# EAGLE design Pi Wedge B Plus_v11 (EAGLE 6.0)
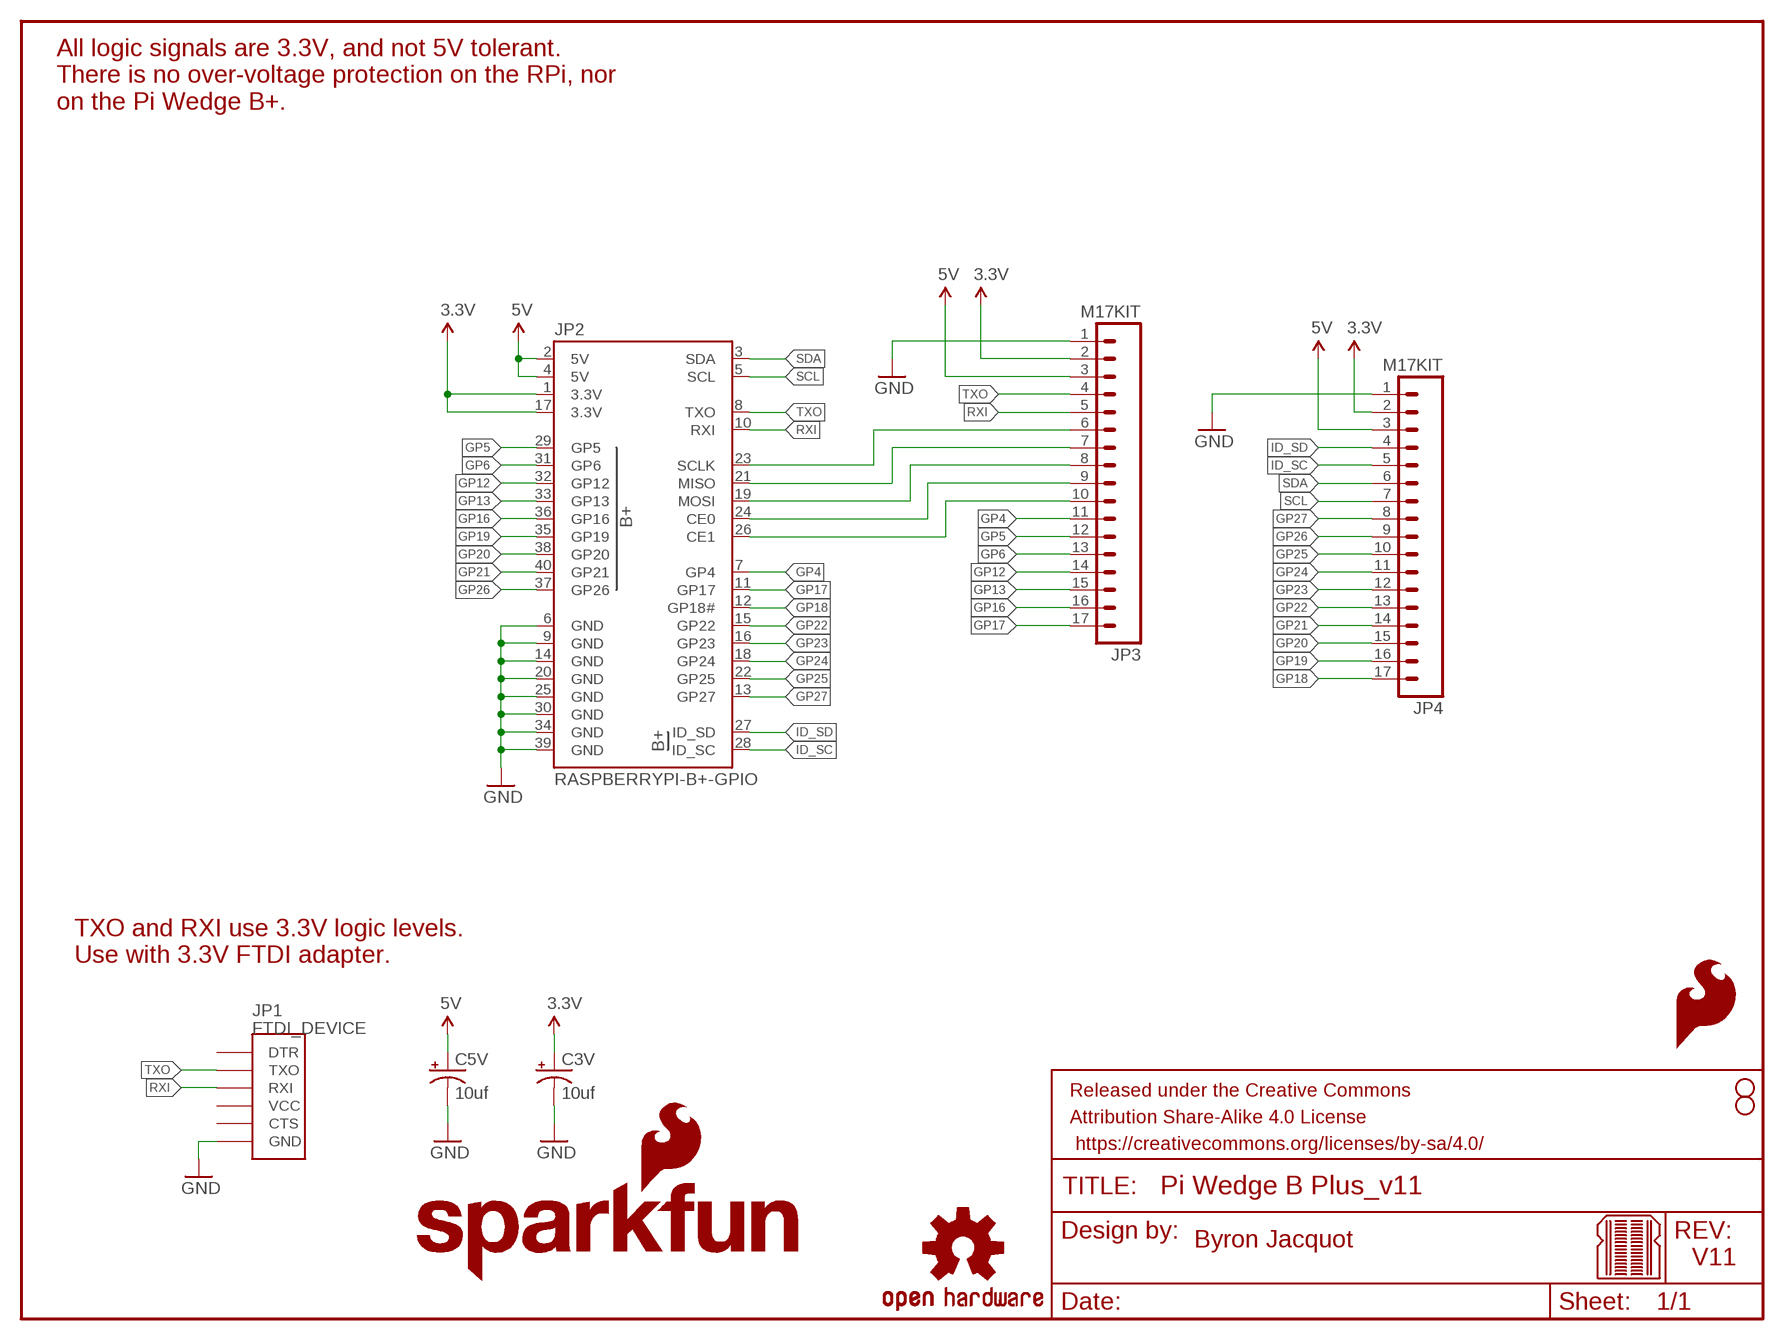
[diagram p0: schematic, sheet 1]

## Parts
C3V  10uf  10UF-25V-20%(PTH)KIT  [CPOL-RADIAL-10UF-25V-KIT]
C5V  10uf  10UF-25V-20%(PTH)KIT  [CPOL-RADIAL-10UF-25V-KIT]
FRAME2  FRAME-LETTER  [CREATIVE_COMMONS]
JP1  FTDI_DEVICE  [FTDI_DEVICE_SIDE]
JP2  RASPBERRYPI-B+-GPIO  [2X20-SHROUDED]
JP3  M17KIT  [1X17_NO_SILK_KIT]
JP4  M17KIT  [1X17_NO_SILK_KIT]
LOGO1  SFE_LOGO_NAME_FLAME.2_INCH  [SFE_LOGO_NAME_FLAME_.2]
LOGO2  SFE_LOGO_NAME_FLAME.2_INCH  [SFE_LOGO_NAME_FLAME_.2]
LOGO3  SFE_LOGO_FLAME.1_INCH  [SFE_LOGO_FLAME_.1]
LOGO4  SFE_LOGO_FLAME.1_INCH  [SFE_LOGO_FLAME_.1]
LOGO5  OSHW-LOGOS  [OSHW-LOGO-S]
STANDOFF1  STAND-OFF  [STAND-OFF]
STANDOFF2  STAND-OFF  [STAND-OFF]
U$2  BREADBOARD_PATTERN  [BREADBOARD_SPACING]

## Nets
3.3V: C3V.1(+) JP2.1(3.3V) JP2.17(3.3V) JP3.2 JP4.2
5V: C5V.1(+) JP2.2(5V) JP2.4(5V) JP3.3 JP4.3
CE0: JP2.24(CE0) JP3.9
CE1: JP2.26(CE1) JP3.10
GND: C3V.2(-) C5V.2(-) JP1.P$6(GND) JP2.6(GND) JP2.9(GND) JP2.14(GND) JP2.20(GND) JP2.25(GND) JP2.30(GND) JP2.34(GND) JP2.39(GND) JP3.1 JP4.1
GP4: JP2.7(GP4) JP3.11
GP5: JP2.29(GP5) JP3.12
GP6: JP2.31(GP6) JP3.13
GP12: JP2.32(GP12) JP3.14
GP13: JP2.33(GP13) JP3.15
GP16: JP2.36(GP16) JP3.16
GP17: JP2.11(GP17) JP3.17
GP18: JP2.12(GP18#) JP4.17
GP19: JP2.35(GP19) JP4.16
GP20: JP2.38(GP20) JP4.15
GP21: JP2.40(GP21) JP4.14
GP22: JP2.15(GP22) JP4.13
GP23: JP2.16(GP23) JP4.12
GP24: JP2.18(GP24) JP4.11
GP25: JP2.22(GP25) JP4.10
GP26: JP2.37(GP26) JP4.9
GP27: JP2.13(GP27) JP4.8
ID_SC: JP2.28(ID_SC) JP4.5
ID_SD: JP2.27(ID_SD) JP4.4
MISO: JP2.21(MISO) JP3.7
MOSI: JP2.19(MOSI) JP3.8
RXI: JP1.P$3(RXI) JP2.10(RXI) JP3.5
SCL: JP2.5(SCL) JP4.7
SCLK: JP2.23(SCLK) JP3.6
SDA: JP2.3(SDA) JP4.6
TXO: JP1.P$2(TXO) JP2.8(TXO) JP3.4
Unconnected: JP1.P$1(DTR) JP1.P$4(VCC) JP1.P$5(CTS)

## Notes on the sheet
- All logic signals are 3.3V, and not 5V tolerant.
  There is no over-voltage protection on the RPi, nor
  on the Pi Wedge B+.
- TXO and RXI use 3.3V logic levels.
  Use with 3.3V FTDI adapter.
- Byron Jacquot
- V11

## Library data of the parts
C3V C5V = SparkFun-Capacitors:10UF-25V-20%(PTH): CAP-08440; PROD_ID: CAP-08440
FRAME2 = SparkFun-Aesthetics:FRAME-LETTER: Schematic Frame
JP1 = SparkFun-Connectors:FTDI_DEVICE: Connector which mates to FTDI basic or FTDI cable.
JP2 = SparkFun-Boards:RASPBERRYPI-B+-GPIO: Raspberry Pi B+ GPIO Header 2x20 pin connector
JP3 JP4 = SparkFun-Connectors:M17: 1x17 .1" header
LOGO1 LOGO2 = SparkFun-Aesthetics:SFE_LOGO_NAME_FLAME: SFE Logo, name and flame
LOGO3 LOGO4 = SparkFun-Aesthetics:SFE_LOGO_FLAME: SFE Logo, flame only
LOGO5 = SparkFun-Aesthetics:OSHW-LOGO: Open Source Hardware Logo This logo indicates the piece of hardware it is found on incorporates a OSHW license and/or adheres to the definition of open source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
STANDOFF1 STANDOFF2 = SparkFun-Electromechanical:STAND-OFF: #4 Stand Off
U$2 = SparkFun-Aesthetics:BREADBOARD_PATTERN: Reference markings that correspond to solderless breadboard row spacing.

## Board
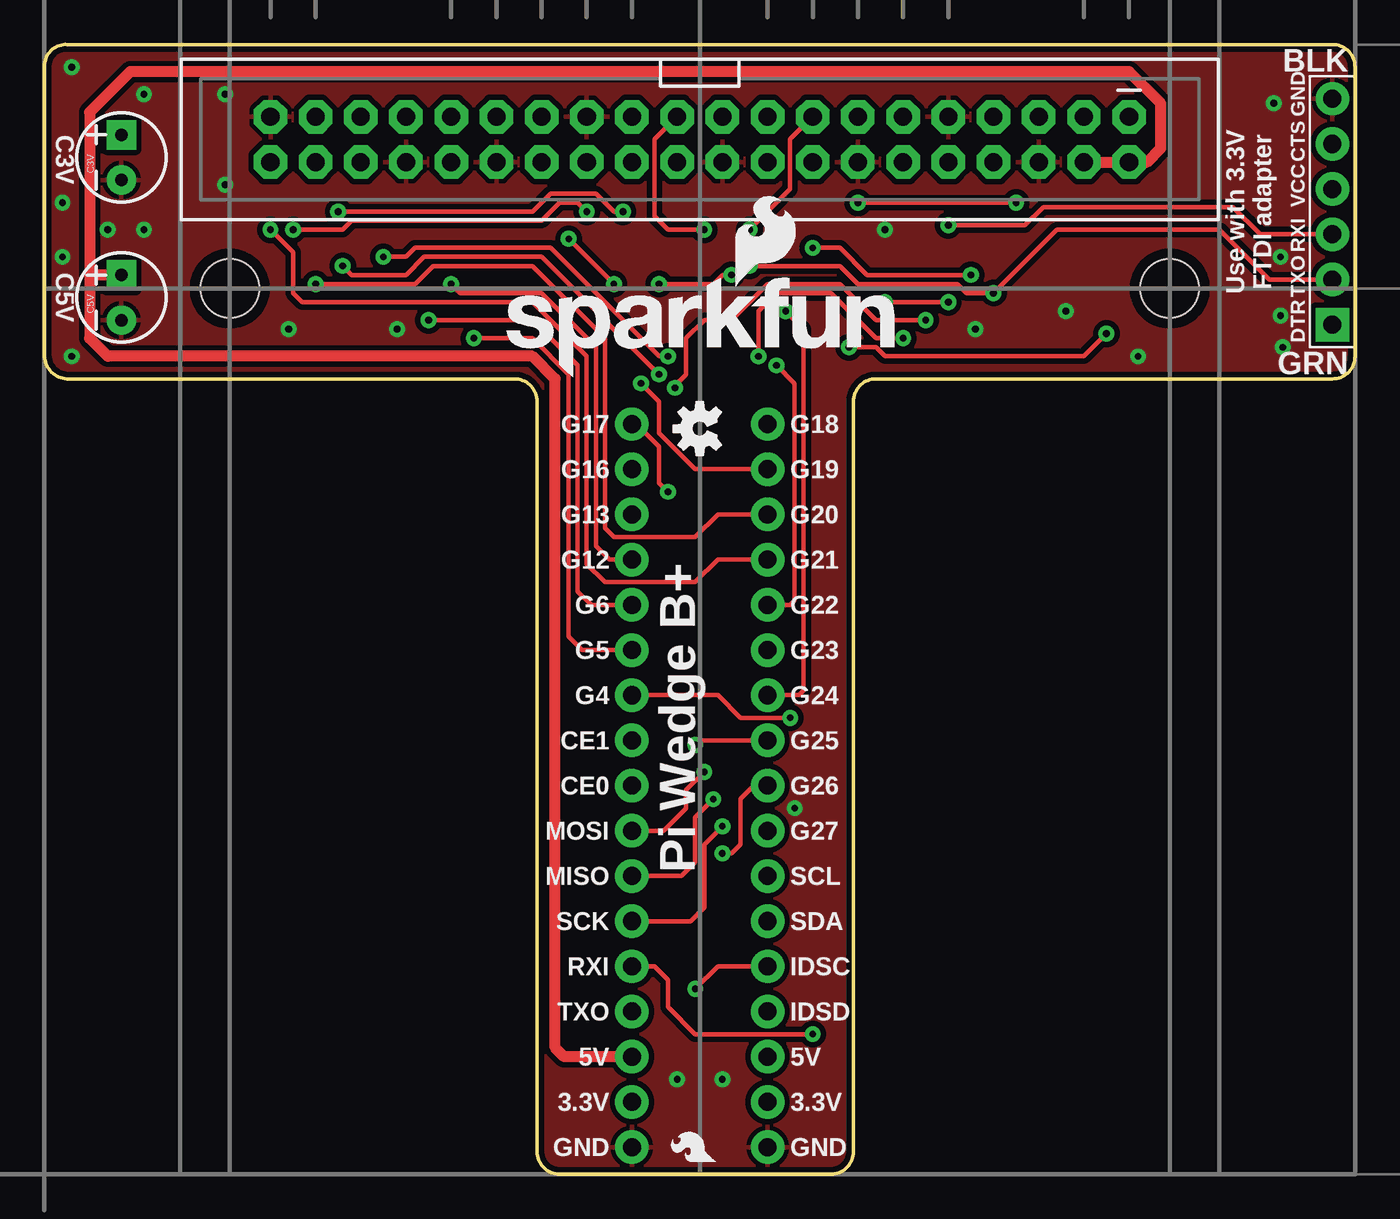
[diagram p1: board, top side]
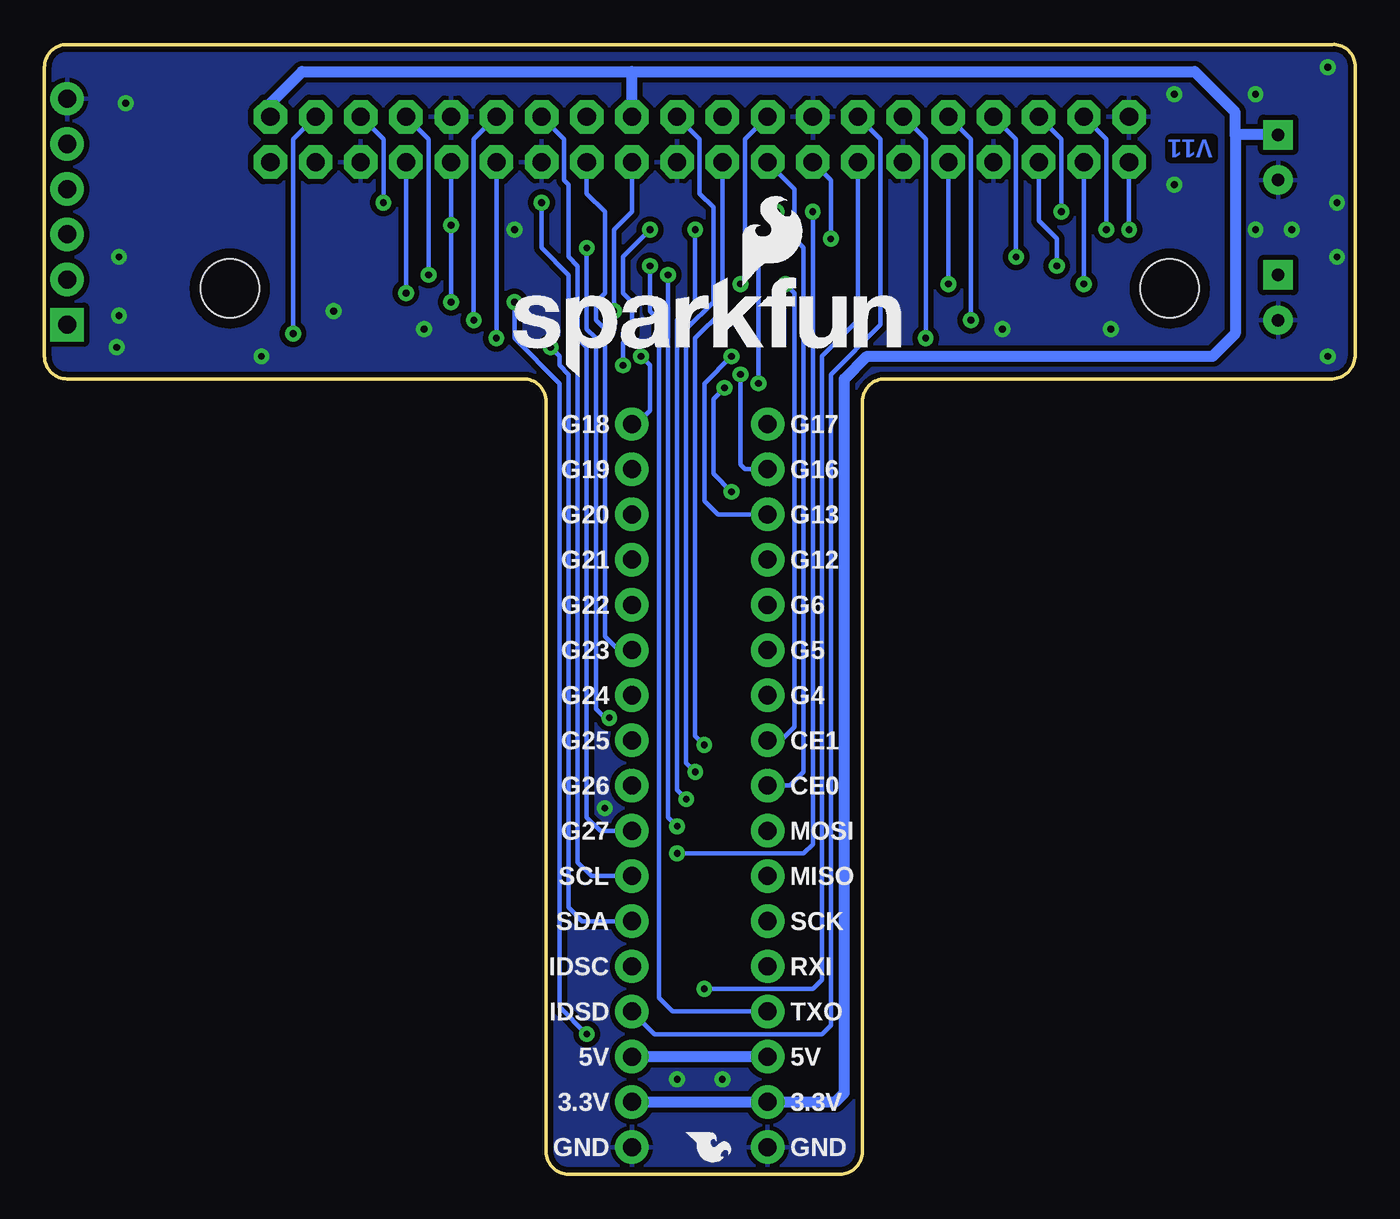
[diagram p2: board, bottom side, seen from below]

Size 73.66 x 63.5 mm. Coordinates in mm from the lower left corner, seen from the top.
Outline: 73.66,62.23 73.66,45.97 arc-90 72.39,44.7 46.74,44.7 arc90 45.47,43.43 45.47,1.27 arc-90 44.2,0 28.96,0 arc-90 27.69,1.27 27.69,43.43 arc90 26.42,44.7 1.27,44.7 arc-90 0,46.1 0,62.36 arc-90 1.27,63.5 72.39,63.5 arc-90 73.66,62.23
Copper layers (1*16): Top 0.035mm / dielectric 1.5mm / Bottom 0.035mm
Design rules "SparkFun-2-layer *": minimum track width 7mil, minimum drill 15mil, track to track 8mil, track to pad 8mil, pad to pad 8mil, via to via 8mil, smd to smd 8mil, copper to edge 8mil, drill to drill 8mil, minimum pad ring 12mil, minimum via ring 10mil, stop-mask expansion 4mil, vias tented up to drill 20mil, thermal gap 10mil

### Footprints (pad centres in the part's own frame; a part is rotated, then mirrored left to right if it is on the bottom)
CPOL-RADIAL-10UF-25V-KIT = drill 0.7 pad 1.651 square: 1 1.27,0 | drill 0.7 pad 1.651: 2 -1.27,0
FTDI_DEVICE_SIDE = drill 1.016 pad 1.88 square: P$1 -6.35,0 | drill 1.016 pad 1.88: P$2 -3.81,0; P$3 -1.27,0; P$4 1.27,0; P$5 3.81,0; P$6 6.35,0
2X20-SHROUDED = drill 1.016 pad 1.88 octagon: 1 -1.27,24.13; 2 1.27,24.13; 3 -1.27,21.59; 4 1.27,21.59; 5 -1.27,19.05; 6 1.27,19.05; 7 -1.27,16.51; 8 1.27,16.51; 9 -1.27,13.97; 10 1.27,13.97; 11 -1.27,11.43; 12 1.27,11.43; 13 -1.27,8.89; 14 1.27,8.89; 15 -1.27,6.35; 16 1.27,6.35; 17 -1.27,3.81; 18 1.27,3.81; 19 -1.27,1.27; 20 1.27,1.27; 21 -1.27,-1.27; 22 1.27,-1.27; 23 -1.27,-3.81; 24 1.27,-3.81; 25 -1.27,-6.35; 26 1.27,-6.35; 27 -1.27,-8.89; 28 1.27,-8.89; 29 -1.27,-11.43; 30 1.27,-11.43; 31 -1.27,-13.97; 32 1.27,-13.97; 33 -1.27,-16.51; 34 1.27,-16.51; 35 -1.27,-19.05; 36 1.27,-19.05; 37 -1.27,-21.59; 38 1.27,-21.59; 39 -1.27,-24.13; 40 1.27,-24.13
1X17_NO_SILK_KIT = drill 1.016 pad 1.88: 1 0,0; 2 2.54,0; 3 5.08,0; 4 7.62,0; 5 10.16,0; 6 12.7,0; 7 15.24,0; 8 17.78,0; 9 20.32,0; 10 22.86,0; 11 25.4,0; 12 27.94,0; 13 30.48,0; 14 33.02,0; 15 35.56,0; 16 38.1,0; 17 40.64,0
STAND-OFF = hole 3.302: 0,0

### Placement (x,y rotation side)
C3V  4.32,57.15 90 top
C5V  4.32,49.28 90 top
FRAME2  not placed on the board
JP1  72.39,54.1 90 top
JP2  36.83,58.17 270 top
JP3  33.02,1.52 90 bottom
JP4  40.64,1.52 90 bottom
LOGO1  25.27,44.7 0 top
LOGO2  48.01,44.7 0 bottom
LOGO3  38.1,0.38 90 top
LOGO4  37.97,2.67 270 bottom
LOGO5  36.83,41.91 90 top
STANDOFF1  10.41,49.78 0 top
STANDOFF2  63.25,49.78 0 top
U$2  36.83,66.29 0 top

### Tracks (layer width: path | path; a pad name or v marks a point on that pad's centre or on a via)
3.3V
  Bottom 0.61: JP4.2 JP3.2 29.21,4.06 28.7,4.57 28.7,44.7 27.43,45.97 8,45.97 6.73,47.24 6.73,58.42 | 40.64,61.98 59.18,61.98 60.96,60.2 JP2.1 | 40.64,61.98 9.02,61.98 6.73,59.69 6.73,58.42 | JP2.17 40.64,61.98 | C3V.1 6.73,58.42
5V
  Top 0.61: JP3.3 29.21,6.6 28.7,7.11 28.7,44.7 27.43,45.97 3.56,45.97 2.54,46.99 2.54,50.55 | JP2.4 JP2.2 61.98,56.9 62.74,57.66 62.74,60.2 60.96,61.98 4.83,61.98 2.54,59.69 2.54,50.55 | C5V.1 2.54,50.55
  Bottom 0.61: JP3.3 JP4.3
CE0
  Bottom 0.254: JP3.9 31.75,21.84 30.99,22.61 30.99,52.07 31.5,52.58 31.5,55.37 JP2.24
CE1  (via drill 0.38)
  Top 0.254: v32,50.04 v29.46,52.58
  Bottom 0.254: JP3.10 32.26,24.38 31.5,25.15 31.5,49.53 v32,50.04 | v29.46,52.58 29.46,55.88 JP2.26
GND  (via drill 0.38)
  other vias: 35.56,5.33 38.1,5.33 69.09,60.2 69.47,48.26 69.6,46.48 61.47,45.97 1.52,62.23 1.02,54.61 1.02,51.56 1.52,45.97 5.59,53.09 5.59,60.71 42.16,20.57 47.24,53.09 69.47,51.56 3.56,53.09 10.16,60.71 10.16,55.63 19.81,47.5 13.72,47.5 57.4,48.51 52.32,47.5
  pour Bottom (isolate 0.305): 1.27,44.7 26.42,44.7 arc-90 27.69,43.43 27.69,1.27 arc90 28.96,0 44.2,0 arc90 45.47,1.27 45.47,43.43 arc-90 46.74,44.7 72.39,44.7 arc90 73.66,45.97 73.66,62.23 arc90 72.39,63.5 1.27,63.5 arc90 0,62.36 0,46.1 arc90
  pour Top (isolate 0.305): 45.47,43.43 45.47,1.27 arc-90 44.2,0 28.96,0 arc-90 27.69,1.27 27.69,43.43 arc90 26.42,44.7 1.27,44.7 arc-90 0,46.1 0,62.36 arc-90 1.27,63.5 72.39,63.5 arc-90 73.66,62.23 73.66,45.97 arc-90 72.39,44.7 46.74,44.7 arc90
GP4  (via drill 0.38)
  Top 0.254: JP3.11 37.85,26.92 39.12,25.65 v41.91,25.65 | v43.18,52.07 44.7,52.07 46.23,50.55 v52.07,50.55
  Bottom 0.254: v41.91,25.65 42.16,25.65 42.67,26.16 42.67,46.99 43.18,47.5 v43.18,52.07 | v52.07,50.55 52.07,58.17 JP2.7
GP5  (via drill 0.38)
  Top 0.254: JP3.12 30.23,29.46 29.46,30.23 29.46,44.96 27.43,46.99 v24.13,46.99
  Bottom 0.254: JP2.29 24.13,58.17 v24.13,46.99
GP6  (via drill 0.38)
  Top 0.254: JP3.13 30.73,32 29.97,32.77 29.97,45.47 27.43,48.01 v21.59,48.01
  Bottom 0.254: JP2.31 21.59,58.17 v21.59,48.01
GP12  (via drill 0.38)
  Top 0.254: JP3.14 31.75,34.54 30.99,35.31 30.99,46.48 27.94,49.53 23.37,49.53 v22.86,50.04
  Bottom 0.254: v22.86,50.04 JP2.32
GP13  (via drill 0.38)
  Top 0.254: v35.05,45.97 34.54,45.97 28.45,52.07 20.83,52.07 20.32,51.56 v19.05,51.56
  Bottom 0.254: JP3.15 35.81,37.08 36.58,37.85 36.58,44.45 v35.05,45.97 | v19.05,51.56 19.05,58.17 JP2.33
GP16  (via drill 0.38)
  Top 0.254: v34.54,44.96 27.94,51.56 21.34,51.56 20.32,50.55 17.27,50.55 v16.76,51.05
  Bottom 0.254: JP3.16 34.29,39.62 34.54,39.88 v34.54,44.96 | v16.76,51.05 16.76,52.58 17.78,53.59 JP2.36
GP17  (via drill 0.38)
  Top 0.254: JP3.17 33.27,42.16 34.54,40.89 34.54,38.86 v35.05,38.35 | v35.43,44.2 35.43,44.32 36.07,44.96 36.07,46.99 37.08,48.01 38.61,48.01 40.64,50.04 44.7,50.04 46.74,48.01 v49.53,48.01
  Bottom 0.254: v35.05,38.35 36.07,39.37 36.07,43.56 v35.43,44.2 | JP2.11 49.53,58.17 v49.53,48.01
GP18  (via drill 0.38)
  Top 0.254: v40.13,45.97 40.13,48.51 41.15,49.53 44.2,49.53 46.74,46.99 v48.26,46.99
  Bottom 0.254: JP4.17 40.39,42.16 39.62,42.93 39.62,45.47 v40.13,45.97 | v48.26,46.99 JP2.12
GP19  (via drill 0.38)
  Top 0.254: JP4.16 36.58,39.62 34.54,41.66 34.54,43.43 v33.53,44.45 | v32.51,54.1 32,54.1 30.99,55.12 28.45,55.12 27.43,54.1 v16.51,54.1
  Bottom 0.254: v33.53,44.45 33.53,51.56 32.51,52.58 v32.51,54.1 | v16.51,54.1 16.51,58.17 JP2.35
GP20  (via drill 0.38)
  Top 0.254: JP4.15 37.85,37.08 36.58,35.81 32,35.81 31.5,36.32 31.5,46.99 27.43,51.05 21.84,51.05 20.83,50.04 v15.24,50.04
  Bottom 0.254: v15.24,50.04 JP2.38
GP21  (via drill 0.38)
  Top 0.254: JP4.14 37.85,34.54 36.58,33.27 31.5,33.27 30.48,34.29 30.48,45.97 27.43,49.02 14.48,49.02 13.97,49.53 13.97,51.82 v12.7,53.09
  Bottom 0.254: v12.7,53.09 JP2.40
GP22  (via drill 0.38)
  Top 0.254: JP4.13 41.91,32 42.16,32.26 42.16,44.45 v41.15,45.47 | v39.62,53.09 41.91,55.37 41.91,58.17 JP2.15
  Bottom 0.254: v41.15,45.47 41.15,46.74 40.64,47.24 40.64,49.02 41.15,49.53 41.15,51.56 v39.62,53.09
GP23
  Bottom 0.254: JP4.12 41.4,29.46 42.16,30.23 42.16,47.5 42.67,48.01 42.67,49.02 42.16,49.53 42.16,54.1 43.18,55.12 JP2.16
GP24  (via drill 0.38)
  Top 0.254: JP4.11 42.42,26.92 42.67,27.18 42.67,47.5 v41.66,48.51
  Bottom 0.254: v41.66,48.51 41.66,53.09 40.64,54.1 JP2.18
GP25  (via drill 0.38)
  Top 0.254: JP4.10 36.83,24.38 v36.58,24.13
  Bottom 0.254: v36.58,24.13 37.08,24.64 37.08,46.99 35.56,48.51 JP2.22
GP26  (via drill 0.38)
  Top 0.254: JP4.9 39.88,21.84 39.12,21.08 39.12,18.54 38.61,18.03 v38.1,18.03 | v30.48,54.1 29.97,54.61 28.96,54.61 27.94,53.59 17.27,53.59 16.76,53.09 v13.97,53.09
  Bottom 0.254: v38.1,18.03 30.99,18.03 30.48,18.54 v30.48,54.1 | JP2.37 13.97,58.17 v13.97,53.09
GP27
  Bottom 0.254: JP4.8 42.42,19.3 43.18,20.07 43.18,46.48 43.69,46.99 43.69,51.05 44.2,51.56 44.2,55.63 44.45,55.88 44.45,58.17 JP2.13
ID_SC  (via drill 0.38)
  Top 0.254: JP4.5 37.85,11.68 v36.58,10.41
  Bottom 0.254: v36.58,10.41 30.48,10.41 29.97,10.92 29.97,45.97 27.94,48.01 JP2.28
ID_SD
  Bottom 0.254: JP4.4 39.37,7.87 29.97,7.87 29.46,8.38 29.46,44.96 26.67,47.75 26.67,58.17 JP2.27
MISO  (via drill 0.38)
  Top 0.254: JP3.7 35.81,16.76 36.58,17.53 36.58,20.07 v37.59,21.08 | v37.08,53.09 35.05,53.09 34.29,53.85 34.29,58.17 JP2.21
  Bottom 0.254: v37.59,21.08 38.1,21.59 38.1,48.01 37.08,49.02 v37.08,53.09
MOSI  (via drill 0.38)
  Top 0.254: JP3.8 34.8,19.3 36.07,20.57 36.07,21.59 v37.08,22.61
  Bottom 0.254: v37.08,22.61 37.59,23.11 37.59,47.5 36.07,49.02 36.07,54.36 36.83,55.12 36.83,58.17 JP2.19
RXI  (via drill 0.38)
  Top 0.254: JP3.5 34.29,11.68 35.05,10.92 35.05,9.4 36.58,7.87 v43.18,7.87 | v47.24,49.02 v50.8,49.02 | JP1.P$3 68.33,52.83 66.8,54.36 56.13,54.36 55.12,53.34 v50.8,53.34
  Bottom 0.254: v43.18,7.87 44.7,9.4 44.7,44.45 47.24,46.99 v47.24,49.02 | v50.8,49.02 v50.8,53.34 JP2.10
SCL  (via drill 0.38)
  Top 0.254: v45.72,54.61 v54.61,54.61
  Bottom 0.254: JP4.7 42.93,16.76 43.69,17.53 43.69,45.97 44.2,46.48 44.2,50.55 45.72,52.07 v45.72,54.61 | v54.61,54.61 54.61,58.17 JP2.5
SCLK  (via drill 0.38)
  Top 0.254: JP3.6 36.32,14.22 37.08,14.99 37.08,18.54 v38.1,19.56 | v34.54,50.04 37.59,50.04 38.1,50.55 v38.61,50.55
  Bottom 0.254: v38.1,19.56 38.61,20.07 v38.61,50.55 | JP2.23 34.29,58.17 34.29,50.29 v34.54,50.04
SDA  (via drill 0.38)
  Top 0.254: v45.21,46.48 46.74,46.48 47.24,45.97 58.42,45.97 v59.69,47.24
  Bottom 0.254: JP2.3 59.69,58.17 v59.69,47.24 | JP4.6 43.43,14.22 44.2,14.99 44.2,44.96 44.7,45.47 44.7,45.97 v45.21,46.48
TXO  (via drill 0.38)
  Top 0.254: JP1.P$2 68.83,50.29 66.04,53.09 56.9,53.09 v53.34,49.53 51.82,49.53 51.31,50.04 45.72,50.04 44.7,51.05 v39.62,51.05
  Bottom 0.254: JP3.4 38.35,9.14 39.12,9.91 39.12,48.01 39.62,48.51 v39.62,51.05 | v53.34,49.53 JP2.8

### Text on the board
Bottom: V11
tPlace: C3V | Use with 3.3V / FTDI adapter | C5V | G17 | G18 | G16 | G19 | G13 | G20 | G12 | G21 | G6 | G22 | G5 | G23 | G4 | G24 | Pi Wedge B+ | CE1 | G25 | CE0 | G26 | MOSI | G27 | MISO | SCL | SCK | SDA | RXI | IDSC | TXO | IDSD | 5V | 5V | 3.3V | 3.3V | GND | GND
bPlace: G17 | G18 | G16 | G19 | G13 | G20 | G12 | G21 | G6 | G22 | G5 | G23 | G4 | G24 | CE1 | G25 | CE0 | G26 | MOSI | G27 | MISO | SCL | SCK | SDA | RXI | IDSC | TXO | IDSD | 5V | 5V | 3.3V | 3.3V | GND | GND
tDocu: Byron Jacquot

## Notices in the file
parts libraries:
SparkFun-Aesthetics: Licensing: CC v3.0 Share-Alike You are welcome to use this library for commercial purposes.
SparkFun-Aesthetics: Released under the Creative Commons Attribution Share-Alike 4.0 License
SparkFun-Aesthetics: https://creativecommons.org/licenses/by-sa/4.0
